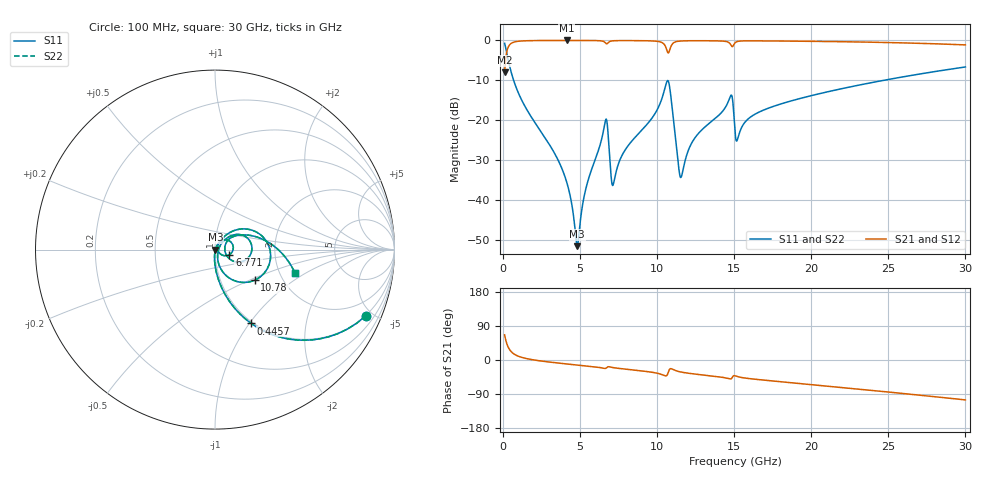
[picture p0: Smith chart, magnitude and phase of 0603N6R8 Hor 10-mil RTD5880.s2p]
# GHz S MA R 50
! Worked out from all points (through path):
!   3201 points, 100 MHz to 30 GHz, reference 50 ohm
!   highest |S21| = -0.02 dB at 4.127 GHz (marker M1); lowest = -8.0 dB at 100 MHz (marker M2)
!   group delay of S21, straight-line fit = 10.4 ps
!   lowest |S11| = -51.6 dB at 4.809 GHz (marker M3), VSWR 1.01, Z = 50.3 - j0.0747 ohm
!   |S11| at or under -10 dB: 682.9 MHz to 24.73 GHz (24.05 GHz wide, 189 % of centre)
!   |S22| runs from -51.6 to -0.7 dB; largest |S21 - S12| = 0
!   S11 on the Smith chart (normalised r, x): 100 MHz: 0.98, -4.59; 445.7 MHz: 0.98, -1.02; 6.771 GHz: 1.17, -0.07; 10.78 GHz: 1.45, -0.54; 30 GHz: 2.42, -0.80
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0.1  0.9182 -23.6  0.396 66.4  0.396 66.4  0.9182 -23.6
0.4457187  0.4586 -63.8  0.888 26.1  0.888 26.1  0.4586 -63.8
1.501562  0.1395 -85.6  0.9889 3.9  0.9889 3.9  0.1395 -85.6
4.127156  0.01673 -92.5  0.9975 -10.4  0.9975 -10.4  0.01673 -92.5
4.80925  0.002624 -16.5  0.9973 -13.2  0.9973 -13.2  0.002624 -16.5
5.089563  0.007083 52.3  0.9971 -14.3  0.9971 -14.3  0.007083 52.3
6.584562  0.08675 37.7  0.9537 -22.3  0.9537 -22.3  0.08675 37.7
6.771438  0.08489 -19.6  0.915 -18.4  0.915 -18.4  0.08489 -19.6
7.014375  0.01931 -22.9  0.9806 -19.1  0.9806 -19.1  0.01931 -22.9
7.163875  0.01592 24.5  0.9885 -20.2  0.9885 -20.2  0.01592 24.5
7.883344  0.04111 58.9  0.9938 -23.8  0.9938 -23.8  0.04111 58.9
10.06978  0.1434 46.1  0.9689 -35.5  0.9689 -35.5  0.1434 46.1
10.77991  0.2799 -37.4  0.7239 -26.1  0.7239 -26.1  0.2799 -37.4
11.53675  0.01907 -11.9  0.9819 -31.7  0.9819 -31.7  0.01907 -11.9
12.37769  0.05715 44.9  0.99 -36.8  0.99 -36.8  0.05715 44.9
14.73231  0.1955 17.2  0.908 -50.1  0.908 -50.1  0.1955 17.2
15.05  0.07228 -26.6  0.9298 -41.6  0.9298 -41.6  0.07228 -26.6
15.21819  0.05775 16.7  0.9701 -43.9  0.9701 -43.9  0.05775 16.7
16.35813  0.119 36.0  0.986 -50.8  0.986 -50.8  0.119 36.0
20.03956  0.2036 23.3  0.973 -65.1  0.973 -65.1  0.2036 23.3
25.01978  0.3238 4.2  0.9391 -84.6  0.9391 -84.6  0.3238 4.2
30  0.4639 -16.3  0.8778 -105.3  0.8778 -105.3  0.4639 -16.3
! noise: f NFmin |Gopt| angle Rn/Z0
0.1  0.0003536  0.9325  0.6008  0.001166
3.417  0.003896  0.8038  9.416  0.004095
6.743  0.03866  0.9578  18.42  0.2013
10.06  0.02128  0.8903  27.3  0.03988
13.39  0.01434  0.796  36.04  0.01316
16.7  0.01499  0.7634  44.55  0.01105
20.03  0.01595  0.74  52.77  0.009918
23.35  0.01809  0.7366  60.81  0.01029
26.67  0.02052  0.7379  68.66  0.0108
30  0.02321  0.7423  76.3  0.01132
